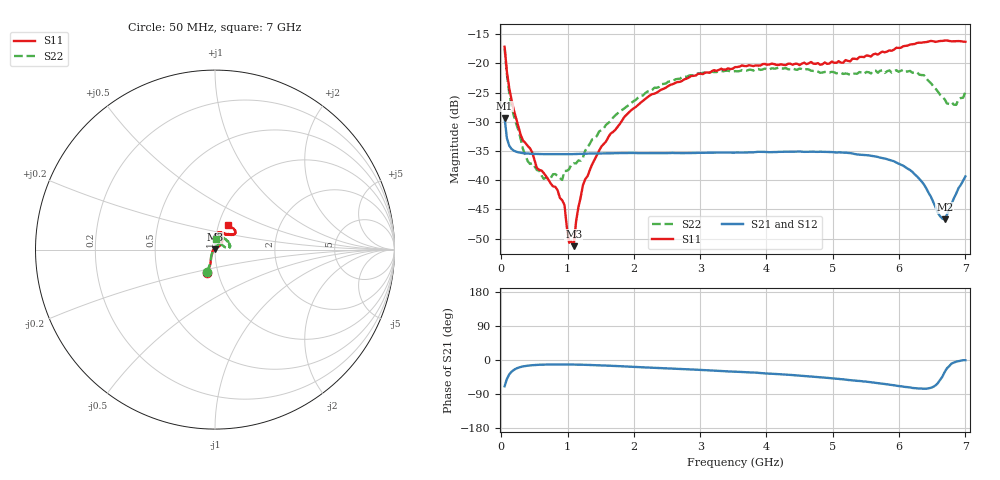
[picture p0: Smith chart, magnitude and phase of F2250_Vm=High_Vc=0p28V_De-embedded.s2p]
! Integrated Device Technology
! Corporate Headquarters
! 6024 Silver Creek Valley Road
! San Jose, CA 95138  USA
! Phone:  1-408-284-8200
! Toll Free:  1-800-223-1366
! Webpage:  http://www.idt.com/
! Timing and RF Division
! 515 Groton Road, Suite 102
! Westford, MA 01886-6024
! Device:  F2250
! Description: Voltage Variable RF Attenuator
! Frequency:  50.0 -  6000.00 MHz
! Package:  3x3 mm Thin QFN Plastic Package: 16 pin
! Ports:  2 RF, 3 DC
!  Pin  1  = GND
!  Pin  2  = NC
!  Pin  3  = RF1  = Port 1
!  Pin  4  = NC
!  Pin  5  = GND
!  Pin  6  = GND
!  Pin  7  = GND
!  Pin  8  = GND
!  Pin  9  = NC
!  Pin 10  = RF2  = Port 2
!  Pin 11  = NC
!  Pin 12  = GND
!  Pin 13  = GND
!  Pin 14  = VCNTRL
!  Pin 15  = VDD
!  Pin 16  = VMODE
! Vcntrl:  0.280 Volts
! Vmode:  +3.300 Volts
! Vdd:  +3.30  Volts
! Current:  1.250 mA
! Data:  The device was measured on a the F2250 evaluation board which has
!  individual transmission lines to the RF pins.  Data was collected
!  using a calibrated network analyzer.  The evaluation board was
!  de-embedded using a TRL calibration technique.
!  The reference plane is the edge of the package pin.
! Misc:  SN 10
!  Action Tracker AT0258
! Date Measured:  2014-11-26
! Date:  2015-10-15  MJV
! Note:
!  Integrated Device Technology supplies this data as a sample of measured
!  data at the package pin for this product.  Your particular data for this
!  product may vary.
!  Data was taken at 25 degrees C.
!  Integrated Device Technology reserves the right to change this data at anytime.
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# GHz S dB R 50
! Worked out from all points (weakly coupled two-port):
!   201 points, 50 MHz to 7 GHz, reference 50 ohm
!   highest |S21| = -29.37 dB at 50 MHz (marker M1); lowest = -46.7 dB at 6.687 GHz (marker M2)
!   lowest |S11| = -51.3 dB at 1.093 GHz (marker M3), VSWR 1.01, Z = 50 + j0.273 ohm
!   |S11| at or under -10 dB: start of sweep to end of sweep
!   |S22| runs from -40.0 to -17.4 dB; largest |S21 - S12| = 5.7e-05
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0.05  -17.18 -108.5  -29.37 -69.3  -29.37 -69.3  -17.42 -110.3
0.08475  -21.47 -107.4  -32.84 -49.9  -32.83 -49.9  -21.95 -108.4
0.15425  -26.23 -116.6  -34.65 -30.9  -34.65 -30.9  -27.25 -119.5
0.29325  -32.28 -127.4  -35.31 -18.4  -35.31 -18.4  -32.97 -131.5
0.3975  -34.12 -142.2  -35.44 -15.0  -35.44 -15.0  -36.70 -156.6
0.5365  -37.90 -154.7  -35.51 -12.9  -35.51 -12.9  -38.26 -179.5
0.64075  -38.78 -162.6  -35.54 -12.2  -35.54 -12.2  -39.77 159.3
0.91875  -43.43 156.4  -35.56 -11.8  -35.56 -11.8  -39.95 123.9
0.9535  -44.25 170.9  -35.56 -11.8  -35.56 -11.8  -38.42 120.4
1.023  -50.69 140.4  -35.55 -11.9  -35.55 -11.9  -38.12 103.7
1.0925  -51.28 89.7  -35.53 -12.0  -35.53 -12.0  -37.12 94.4
1.12725  -47.13 61.4  -35.52 -12.2  -35.52 -12.2  -37.13 87.4
1.2315  -40.86 40.7  -35.49 -12.5  -35.48 -12.5  -36.15 73.1
1.6485  -32.02 41.2  -35.40 -15.2  -35.40 -15.3  -29.90 57.9
2.37825  -24.76 46.7  -35.36 -21.1  -35.36 -21.1  -24.04 52.9
3.525  -20.66 71.7  -35.28 -30.7  -35.29 -30.8  -21.34 72.4
4.7065  -20.06 72.0  -35.12 -44.0  -35.13 -44.0  -21.30 70.0
5.85325  -17.79 40.5  -36.55 -65.0  -36.55 -65.1  -21.20 22.9
6.27025  -16.53 39.4  -39.34 -74.6  -39.35 -74.6  -21.52 8.1
6.68725  -16.11 47.9  -46.71 -31.9  -46.70 -31.5  -26.16 28.0
6.861  -16.22 54.5  -42.31 -4.3  -42.25 -4.3  -27.11 57.5
7  -16.32 62.4  -39.35 -0.6  -39.32 -0.8  -24.91 84.0
